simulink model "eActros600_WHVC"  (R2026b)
undefined symbols (not defined in the file or in its folder): DiscIntNeverNeededParam

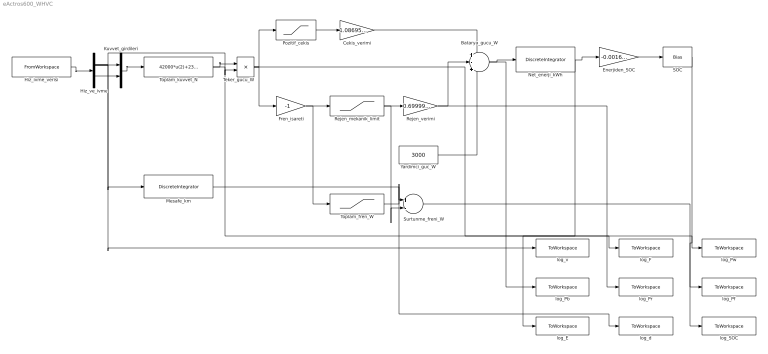
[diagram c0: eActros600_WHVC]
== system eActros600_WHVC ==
  Batarya_gucu_W : Sum  Inputs=+-+
  Cekis_verimi : Gain  Gain=1.0869565217391304
  Enerjiden_SOC : Gain  Gain=-0.0016666666666666668
  Fren_isareti : Gain  Gain=-1
  Hiz_ivme_verisi : FromWorkspace  VariableName=girdi  SampleTime=1  Interpolate=off  OutputAfterFinalValue=Holding final value
  Hiz_ve_ivme : Demux  Outputs=2
  Kuvvet_girdileri : Mux  Inputs=2
  Mesafe_km : DiscreteIntegrator  IntegratorMethod=Integration: Trapezoidal  gainval=0.001  ICPrevOutput=DiscIntNeverNeededParam  ICPrevScaledInput=DiscIntNeverNeededParam
  Net_enerji_kWh : DiscreteIntegrator  IntegratorMethod=Integration: Trapezoidal  gainval=2.7777777777777776e-07  ICPrevOutput=DiscIntNeverNeededParam  ICPrevScaledInput=DiscIntNeverNeededParam
  Pozitif_cekis : Saturate  UpperLimit=inf  LowerLimit=0
  Rejen_mekanik_limit : Saturate  UpperLimit=300000  LowerLimit=0
  Rejen_verimi : Gain  Gain=0.69999999999999996
  SOC : Bias  Bias=0.80000000000000004
  Surtunme_freni_W : Sum  Inputs=+-
  Teker_gucu_W : Product
  Toplam_fren_W : Saturate  UpperLimit=inf  LowerLimit=0
  Toplam_kuvvet_N : Fcn  Expr=42000*u(2)+2354.4000000000001*(u(1)>0)+3.6749999999999998*u(1)^2+0
  Yardimci_guc_W : Constant  Value=3000
  log_E : ToWorkspace  VariableName=log_E  SaveFormat=Timeseries  SampleTime=-1
  log_F : ToWorkspace  VariableName=log_F  SaveFormat=Timeseries  SampleTime=-1
  log_Pb : ToWorkspace  VariableName=log_Pb  SaveFormat=Timeseries  SampleTime=-1
  log_Pf : ToWorkspace  VariableName=log_Pf  SaveFormat=Timeseries  SampleTime=-1
  log_Pr : ToWorkspace  VariableName=log_Pr  SaveFormat=Timeseries  SampleTime=-1
  log_Pw : ToWorkspace  VariableName=log_Pw  SaveFormat=Timeseries  SampleTime=-1
  log_SOC : ToWorkspace  VariableName=log_SOC  SaveFormat=Timeseries  SampleTime=-1
  log_d : ToWorkspace  VariableName=log_d  SaveFormat=Timeseries  SampleTime=-1
  log_v : ToWorkspace  VariableName=log_v  SaveFormat=Timeseries  SampleTime=-1
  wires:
  Hiz_ivme_verisi/1 -> Hiz_ve_ivme/1
  Hiz_ve_ivme/1 -> Kuvvet_girdileri/1, Teker_gucu_W/2, Mesafe_km/1, log_v/1
  Hiz_ve_ivme/2 -> Kuvvet_girdileri/2
  Kuvvet_girdileri/1 -> Toplam_kuvvet_N/1
  Toplam_kuvvet_N/1 -> Teker_gucu_W/1, log_F/1
  Teker_gucu_W/1 -> Pozitif_cekis/1, Fren_isareti/1, log_Pw/1
  Pozitif_cekis/1 -> Cekis_verimi/1
  Fren_isareti/1 -> Rejen_mekanik_limit/1, Toplam_fren_W/1
  Rejen_mekanik_limit/1 -> Rejen_verimi/1, Surtunme_freni_W/2
  Cekis_verimi/1 -> Batarya_gucu_W/1
  Rejen_verimi/1 -> Batarya_gucu_W/2, log_Pr/1
  Yardimci_guc_W/1 -> Batarya_gucu_W/3
  Batarya_gucu_W/1 -> Net_enerji_kWh/1, log_Pb/1
  Net_enerji_kWh/1 -> Enerjiden_SOC/1, log_E/1
  Enerjiden_SOC/1 -> SOC/1
  Toplam_fren_W/1 -> Surtunme_freni_W/1
  Surtunme_freni_W/1 -> log_Pf/1
  Mesafe_km/1 -> log_d/1
  SOC/1 -> log_SOC/1
